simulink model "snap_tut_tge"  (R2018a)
settings: Solver=VariableStepDiscrete  StartTime=0.0  StopTime=50000  RelTol=1e-3
undefined symbols (not defined in the file): bad_frame, Bit, Both, bram, c, cnt_rst, core_rst, d, data, data_in, eof, eof_in, Falling, hex2dec, ip, ip_in, led, led_rx, led_tx, led_up, link_up, Location, Lower, Minimum_Area, notused, out, overrun, reg, Rising, ROACH2, sfp, SNAP, tx_full, tx_over, Unsigned, Upper, valid, valid_in, Width, xc7k160t
libraries: xbsIndex_r4 x1201, casper_library_misc x9, xps_library x5
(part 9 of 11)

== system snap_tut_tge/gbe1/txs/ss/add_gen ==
  note: Force MSbit of count to be '1' by negating busy as counter bit may be '0' or '1'
  note: A total count of bytes written to BRAM since trig
  note: Count of bytes in BRAM as well as done signal
  note: Do one capture by default
  note: prevent one extra write to address 0
  note: To storage
  vin : Inport
  din : Inport  Port=2
  we : Inport  Port=3
  go : Inport  Port=4
  cont : Inport  Port=5
  init : Inport  Port=6
  Concat : xbsIndex_r4/Concat  num_inputs=3  dbl_ovrd=off  block_type=concat
  Convert : xbsIndex_r4/Convert  gui_display_data_type=Fixed-point  arith_type=Unsigned  n_bits=32-nsamples-log2(increment)-1  bin_pt=0  float_type=Single  exp_bits=8  fraction_bits=24  quantization=Truncate  overflow=Wrap  en=off  latency=0  pipeline=off  dbl_ovrd=off  block_type=convert
  Delay{,3..6} (5 alike) : xbsIndex_r4/Delay  rst=off  infoeditControl=Selection of Reset will increase slice count due to use of real FFs and instead of SRLs  en=off  latency=1  reg_retiming=on  dbl_ovrd=off  block_type=delay
  Delay1 : xbsIndex_r4/Delay  rst=off  infoeditControl=Selection of Reset will increase slice count due to use of real FFs and instead of SRLs  en=off  latency=1  reg_retiming=off  dbl_ovrd=off  block_type=delay
  Delay2 : xbsIndex_r4/Delay  rst=off  infoeditControl=Selection of Reset will increase slice count due to use of real FFs and instead of SRLs  en=off  latency=1  reg_retiming=off  dbl_ovrd=off  block_type=delay
  Delay7 : xbsIndex_r4/Delay  rst=off  infoeditControl=Selection of Reset will increase slice count due to use of real FFs and instead of SRLs  en=off  latency=1  reg_retiming=off  dbl_ovrd=off  block_type=delay
  Inverter : xbsIndex_r4/Inverter  en=off  latency=1  dbl_ovrd=off  block_type=inv
  Inverter1 : xbsIndex_r4/Inverter  en=off  latency=0  dbl_ovrd=off  block_type=inv
  Logical1 : xbsIndex_r4/Logical  logical_function=AND  inputs=2  en=off  latency=1  precision=Full  arith_type=Unsigned  n_bits=8  bin_pt=2  align_bp=on  dbl_ovrd=off  block_type=logical
  Logical2 : xbsIndex_r4/Logical  logical_function=AND  inputs=2  en=off  latency=1  precision=Full  arith_type=Unsigned  n_bits=8  bin_pt=2  align_bp=on  dbl_ovrd=off  block_type=logical
  Logical4 : xbsIndex_r4/Logical  logical_function=OR  inputs=2  en=off  latency=0  precision=Full  arith_type=Unsigned  n_bits=8  bin_pt=2  align_bp=on  dbl_ovrd=off  block_type=logical
  Logical6 : xbsIndex_r4/Logical  logical_function=AND  inputs=3  en=off  latency=0  precision=Full  arith_type=Unsigned  n_bits=8  bin_pt=2  align_bp=on  dbl_ovrd=off  block_type=logical
  Register3 : xbsIndex_r4/Register  init=0  rst=on  en=on  dbl_ovrd=off  block_type=register
  Register4 : xbsIndex_r4/Register  init=0  rst=off  en=on  dbl_ovrd=off  block_type=register
  Register5 : xbsIndex_r4/Register  init=1  rst=on  en=on  dbl_ovrd=off  block_type=register
  Shift : xbsIndex_r4/Shift  shift_dir=Left  shift_bits=32-nsamples-log2(increment)-1-1  en=off  latency=1  precision=Full  arith_type="Signed  (2's comp)"  n_bits=16  bin_pt=14  quantization=Truncate  overflow=Wrap  dbl_ovrd=off  block_type=shift
  add_gen : xbsIndex_r4/Counter  cnt_type=Free Running  cnt_to=1  operation=Up  start_count=0  cnt_by_val=increment  arith_type=Unsigned  n_bits=counter_size  bin_pt=0  load_pin=off  rst=on  en=on  explicit_period=on  period=1  use_behavioral_HDL=off  implementation=DSP48  use_rpm=on  dbl_ovrd=off  block_type=counter
  edge_detect : Subsystem  AncestorBlock=casper_library_misc/edge_detect  mask(edge_detect){edge=Both, polarity=Active High, x_in=[0 0.08 0.08 0.16 0.16 0.24 0.24 0.32 0.32 0.4], y_in=[-1 -1  1  1  1  1 -1 -1 -1 -1], x_out=[0.6 0.68 0.68 0.76 0.76 0.84 0.84 0.92 0.92 1], y_out=[-1 -1  1  1 -1 -1  1  1 -1 -1]}
      mask prompts: edge "Edge Type"; polarity "Output Polarity"; x_in "Input X Positions"; y_in "Input Y Positions"; x_out "Output X Positions"; y_out "Output Y Positions"
      mask help: Output is active for one-cycle after each edge of the specified type (i.e. rising, falling or both).
      mask init:
      | edge_detect_init(gcb,...
      |     'edge',edge,...
      |     'polarity',polarity,...
      |     'x_in',x_in,...
      |     'x_out',x_out,...
      |     'y_in',y_in,...
      |     'y_out',y_out);
      | 
      | x_in_num=str2num(getfield(getfield(get_param(gcb,'UserData'),'parameters'),'x_in'));
      | x_out_num=str2num(getfield(getfield(get_param(gcb,'UserData'),'parameters'),'x_out'));
      | y_in_num=str2num(getfield(getfield(get_param(gcb,'UserData'),'parameters'),'y_in'));
      | y_out_num=str2num(getfield(getfield(get_param(gcb,'UserData'),'parameters'),'y_out'));
  edge_detect1 : Subsystem  AncestorBlock=casper_library_scopes/snapshot/add_gen/edge_detect  mask(edge_detect){edge=Both, polarity=Active High, x_in=[0 0.08 0.08 0.16 0.16 0.24 0.24 0.32 0.32 0.4], y_in=[-1 -1  1  1  1  1 -1 -1 -1 -1], x_out=[0.6 0.68 0.68 0.76 0.76 0.84 0.84 0.92 0.92 1], y_out=[-1 -1  1  1 -1 -1  1  1 -1 -1]}
      mask prompts: edge "Edge Type"; polarity "Output Polarity"; x_in "Input X Positions"; y_in "Input Y Positions"; x_out "Output X Positions"; y_out "Output Y Positions"
      mask help: Output is active for one-cycle after each edge of the specified type (i.e. rising, falling or both).
      mask init:
      | edge_detect_init(gcb,...
      |     'edge',edge,...
      |     'polarity',polarity,...
      |     'x_in',x_in,...
      |     'x_out',x_out,...
      |     'y_in',y_in,...
      |     'y_out',y_out);
      | 
      | x_in_num=str2num(getfield(getfield(get_param(gcb,'UserData'),'parameters'),'x_in'));
      | x_out_num=str2num(getfield(getfield(get_param(gcb,'UserData'),'parameters'),'x_out'));
      | y_in_num=str2num(getfield(getfield(get_param(gcb,'UserData'),'parameters'),'y_in'));
      | y_out_num=str2num(getfield(getfield(get_param(gcb,'UserData'),'parameters'),'y_out'));
  slice1 : xbsIndex_r4/Slice  nbits=nsamples+log2(increment)  boolean_output=off  mode=Lower Bit Location + Width  bit1=0  base1=LSB of Input  bit0=0  base0=LSB of Input  dbl_ovrd=off  block_type=slice
  slice2 : xbsIndex_r4/Slice  nbits=nsamples-burst_size  boolean_output=off  mode=Lower Bit Location + Width  bit1=0  base1=LSB of Input  bit0=log2(increment)+burst_size  base0=LSB of Input  dbl_ovrd=off  block_type=slice
  slice3 : xbsIndex_r4/Slice  nbits=1  boolean_output=on  mode=Lower Bit Location + Width  bit1=0  base1=MSB of Input  bit0=nsamples + log2(increment)  base0=LSB of Input  dbl_ovrd=off  block_type=slice
  vout : Outport
  add : Outport  Port=2
  dout : Outport  Port=3
  we_o : Outport  Port=4
  status : Outport  Port=5
  en_cnt : Outport  Port=6
  done : Outport  Port=7
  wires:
  Delay6/1 -> dout/1
  Delay5/1 -> Delay7/1
  Delay4/1 -> Delay/1, Register3/1, Register3/3, add_gen/1
  Delay3/1 -> Register5/1, Logical4/1
  Delay7/1 -> Register4/1
  Logical1/1 -> Logical6/3
  go/1 -> Logical1/2
  we/1 -> Logical1/1
  Logical4/1 -> Logical6/2
  Inverter/1 -> Concat/2
  slice1/1 -> Delay1/1
  Delay1/1 -> Concat/3
  din/1 -> Delay6/1
  Delay2/1 -> en_cnt/1
  slice2/1 -> add/1
  Convert/1 -> Shift/1
  Concat/1 -> status/1
  Logical6/1 -> add_gen/2, Register3/2, Logical2/1, we_o/1
  init/1 -> Delay4/1
  slice3/1 -> edge_detect/1(in)
  Register5/1 -> Logical6/1, edge_detect1/1(in), Inverter/1, Convert/1
  add_gen/1 -> slice3/1, Delay2/1, slice1/1, slice2/1
  vin/1 -> Delay5/1
  Register3/1 -> Logical2/2
  Logical2/1 -> Register4/2
  Register4/1 -> vout/1
  edge_detect/1(out) -> Register5/3, Inverter1/1
  cont/1 -> Delay3/1
  Inverter1/1 -> Logical4/2
  Delay/1 -> Register5/2
  Shift/1 -> Concat/1
  edge_detect1/1(out) -> done/1

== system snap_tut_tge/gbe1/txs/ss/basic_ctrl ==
  vin : Inport
  din : Inport  Port=2
  we : Inport  Port=3
  trig : Inport  Port=4
  ctrl : Inport  Port=5
  stopi : Inport  Port=6
  Constant : xbsIndex_r4/Constant  const=1  gui_display_data_type=Fixed-point  arith_type=Boolean  n_bits=16  bin_pt=14  preci_type=Single  exp_width=8  frac_width=24  explicit_period=on  period=1  equ=P=C  opselect=C  inp2=PCIN>>17  opr=+  inp1=P  carry=CIN  dbl_ovrd=off  block_type=constant
  Constant1 : xbsIndex_r4/Constant  const=1  gui_display_data_type=Fixed-point  arith_type=Boolean  n_bits=1  bin_pt=0  preci_type=Single  exp_width=8  frac_width=24  explicit_period=on  period=1  equ=P=C  opselect=C  inp2=PCIN>>17  opr=+  inp1=P  carry=CIN  dbl_ovrd=off  block_type=constant
  Constant2 : xbsIndex_r4/Constant  const=1  gui_display_data_type=Fixed-point  arith_type=Boolean  n_bits=1  bin_pt=0  preci_type=Single  exp_width=8  frac_width=24  explicit_period=on  period=1  equ=P=C  opselect=C  inp2=PCIN>>17  opr=+  inp1=P  carry=CIN  dbl_ovrd=off  block_type=constant
  Delay1 : xbsIndex_r4/Delay  rst=off  infoeditControl=Selection of Reset will increase slice count due to use of real FFs and instead of SRLs  en=off  latency=1  reg_retiming=off  dbl_ovrd=off  block_type=delay
  Delay2 : xbsIndex_r4/Delay  rst=off  infoeditControl=Selection of Reset will increase slice count due to use of real FFs and instead of SRLs  en=off  latency=1  reg_retiming=off  dbl_ovrd=off  block_type=delay
  Delay3 : xbsIndex_r4/Delay  rst=off  infoeditControl=Selection of Reset will increase slice count due to use of real FFs and instead of SRLs  en=off  latency=1  reg_retiming=off  dbl_ovrd=off  block_type=delay
  Inverter : xbsIndex_r4/Inverter  en=off  latency=0  dbl_ovrd=off  block_type=inv
  Logical : xbsIndex_r4/Logical  logical_function=AND  inputs=2  en=off  latency=0  precision=Full  arith_type=Unsigned  n_bits=16  bin_pt=0  align_bp=on  dbl_ovrd=off  block_type=logical
  Mux1 : xbsIndex_r4/Mux  inputs=2  en=off  latency=0  precision=Full  arith_type="Signed  (2's comp)"  n_bits=8  bin_pt=2  quantization=Truncate  overflow=Wrap  dbl_ovrd=off  block_type=mux
  Mux2 : xbsIndex_r4/Mux  inputs=2  en=off  latency=0  precision=Full  arith_type="Signed  (2's comp)"  n_bits=8  bin_pt=2  quantization=Truncate  overflow=Wrap  dbl_ovrd=off  block_type=mux
  Register1 : xbsIndex_r4/Register  init=0  rst=on  en=on  dbl_ovrd=off  block_type=register
  Register6 : xbsIndex_r4/Register  init=0  rst=on  en=on  dbl_ovrd=off  block_type=register
  dram_munge : Subsystem  mask{dram=off, data_width=data_width}
      mask prompts: data_width "data width"
      mask init:
      | set_param(gcb,'LinkStatus','inactive');
      | if strcmp(dram,'on'),
      |     set_param([gcb,'/dram'], 'const', '1');
      | else,
      |     set_param([gcb,'/dram'], 'const', '0');
      | end
      | set_param([gcb,'/data_choice'], ...
      |         'precision', 'User Defined', ...
      |         'arith_type', 'Unsigned', ...
      |         'n_bits', num2str(data_width), 'bin_pt', '0', ...
      |         'quantization', 'Truncate', ...
      |         'overflow', 'Wrap');
  edge_detect : casper_library_misc/edge_detect  edge=Rising  polarity=Active High  x_in=[0 0.08 0.08 0.16 0.16 0.24 0.24 0.32 0.32 0.4]  y_in="[-1 -1  1  1  1  1  1  1  1  1]"  x_out=[0.6 0.68 0.68 0.76 0.76 0.84 0.84 0.92 0.92 1]  y_out="[-1 -1  1  1 -1 -1 -1 -1 -1 -1]"
      link override Delay: sg_icon_stat=45,16,1,1,white,blue,0,07b98262,right,,[ ],[ ]  sg_mask_display=fprintf('','COMMENT: begin icon graphics'); patch([0 45 45 0 0 ],[0 0 16 16 0 ],[0.77 0.82 0.91 ]); plot([0 45 45 0 0 ],[0 0 16 16 0 ]); patch([17.55 20.44 22.44 24.44 26.44 22.44 19.55 17.55 ],[10.22 10.22 12.22 10.22 12.22 12.22 12.22 10.22 ],[1 1 1 ]); patch([19.55 22.44 20.44 17.55 19.55 ],[8.22 8.22 10.22 10.22 8.22 ],[0.931 0.946 0.973 ]); patch([17.55 20.44 22.44 19.55 17.55 ],[6.22 6.22 8.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
      link override Inverter: sg_icon_stat=45,16,1,1,white,blue,0,267846e5,right,,[ ],[ ]  sg_mask_display=fprintf('','COMMENT: begin icon graphics'); patch([0 45 45 0 0 ],[0 0 16 16 0 ],[0.77 0.82 0.91 ]); plot([0 45 45 0 0 ],[0 0 16 16 0 ]); patch([17.55 20.44 22.44 24.44 26.44 22.44 19.55 17.55 ],[10.22 10.22 12.22 10.22 12.22 12.22 12.22 10.22 ],[1 1 1 ]); patch([19.55 22.44 20.44 17.55 19.55 ],[8.22 8.22 10.22 10.22 8.22 ],[0.931 0.946 0.973 ]); patch([17.55 20.44 22.44 19.55 17.55 ],[6.22 6.22 8.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
      link override edge_op: sg_icon_stat=45,44,2,1,white,blue,0,affe8783,right,,[ ],[ ]  sg_mask_display=fprintf('','COMMENT: begin icon graphics'); patch([0 45 45 0 0 ],[0 0 44 44 0 ],[0.77 0.82 0.91 ]); plot([0 45 45 0 0 ],[0 0 44 44 0 ]); patch([8.65 17.32 23.32 29.32 35.32 23.32 14.65 8.65 ],[28.66 28.66 34.66 28.66 34.66 34.66 34.66 28.66 ],[1 1 1 ]); patch([14.65 23.32 17.32 8.65 14.65 ],[22.66 22.66 28.66 28.66 22.66 ],[0.931 0.946 0.973 ]); patch([8.65 17.32 23.32 14.65 8.65 ],[16.66 16.66 22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
  enable : xbsIndex_r4/Slice  nbits=1  boolean_output=on  mode=Lower Bit Location + Width  bit1=0  base1=LSB of Input  bit0=0  base0=LSB of Input  dbl_ovrd=off  block_type=slice
  trig_src : xbsIndex_r4/Slice  nbits=1  boolean_output=on  mode=Lower Bit Location + Width  bit1=0  base1=LSB of Input  bit0=1  base0=LSB of Input  dbl_ovrd=off  block_type=slice
  valid_src : xbsIndex_r4/Slice  nbits=1  boolean_output=on  mode=Lower Bit Location + Width  bit1=0  base1=LSB of Input  bit0=2  base0=LSB of Input  dbl_ovrd=off  block_type=slice
  vout : Outport
  dout : Outport  Port=2
  we_o : Outport  Port=3
  go : Outport  Port=4
  stop : Outport  Port=5
  init : Outport  Port=6
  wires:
  Delay1/1 -> edge_detect/1
  Delay3/1 -> Mux1/1
  Delay2/1 -> Mux2/1
  dram_munge/1(vout) -> vout/1
  vin/1 -> dram_munge/1(vin)
  dram_munge/3(we_o) -> we_o/1
  dram_munge/2(dout) -> dout/1
  din/1 -> dram_munge/2(din)
  Inverter/1 -> Logical/2
  Mux2/1 -> Logical/1, Register6/1
  Register6/1 -> go/1
  trig/1 -> Mux2/2
  Mux1/1 -> dram_munge/3(we)
  we/1 -> Mux1/2
  ctrl/1 -> enable/1, valid_src/1, trig_src/1
  edge_detect/1 -> Inverter/1, Register1/3, dram_munge/4(init), Register6/2, init/1
  enable/1 -> Delay1/1
  Constant1/1 -> Mux2/3
  Constant2/1 -> Mux1/3
  trig_src/1 -> Delay2/1
  valid_src/1 -> Delay3/1
  Constant/1 -> Register1/1
  Register1/1 -> Register6/3
  Logical/1 -> Register1/2
  stopi/1 -> stop/1

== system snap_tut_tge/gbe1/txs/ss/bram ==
  addr : Inport
  data_in : Inport  Port=2
  we : Inport  Port=3
  Terminator : Terminator
  Terminator1 : Terminator
  Terminator2 : Terminator
  calc_add : Subsystem  mask{data_width=128, addr_width=13, sample_rate=sample_rate}
      mask prompts: data_width "data width"; addr_width "address width"; sample_rate "sample rate"
  convert_addr : xbsIndex_r4/Convert  gui_display_data_type=Fixed-point  arith_type=Unsigned  n_bits=addr_width  bin_pt=0  float_type=Single  exp_bits=8  fraction_bits=24  quantization=Truncate  overflow=Wrap  en=off  latency=0  pipeline=off  dbl_ovrd=off  block_type=convert
  convert_din1 : xbsIndex_r4/Convert  gui_display_data_type=Fixed-point  arith_type=Unsigned  n_bits=128  bin_pt=0  float_type=Single  exp_bits=8  fraction_bits=24  quantization=Truncate  overflow=Wrap  en=off  latency=0  pipeline=off  dbl_ovrd=off  block_type=convert
  convert_we : xbsIndex_r4/Convert  gui_display_data_type=Fixed-point  arith_type=Unsigned  n_bits=1  bin_pt=0  float_type=Single  exp_bits=8  fraction_bits=24  quantization=Truncate  overflow=Wrap  en=off  latency=0  pipeline=off  dbl_ovrd=off  block_type=convert
  munge_in : Subsystem  AncestorBlock=casper_library_flow_control/munge  mask(munge){divisions=4, div_size=[32 32 32 32], order=[3  2  1  0], arith_type_out=Unsigned, bin_pt_out=0}
      mask prompts: divisions "Number of divisions"; div_size "Division size (bits)"; order "Division packing order"; arith_type_out "Output arithmetic type"; bin_pt_out "Output binary point"
      mask help: Splits an input bus into the specified number of divisions and then recombines them in the order specified (most significant division = 0,least = number divisions-1)
      mask init:
      | munge_init(gcb, ...
      |     'divisions', divisions, ...
      |     'div_size', div_size, ...
      |     'order', order, ...
      |     'arith_type_out', arith_type_out, ...
      |     'bin_pt_out', bin_pt_out);
  munge_out : Subsystem  AncestorBlock=casper_library_flow_control/munge  mask(munge){divisions=4, div_size=[32 32 32 32], order=[3  2  1  0], arith_type_out=Unsigned, bin_pt_out=0}
      mask prompts: divisions "Number of divisions"; div_size "Division size (bits)"; order "Division packing order"; arith_type_out "Output arithmetic type"; bin_pt_out "Output binary point"
      mask help: Splits an input bus into the specified number of divisions and then recombines them in the order specified (most significant division = 0,least = number divisions-1)
      mask init:
      | munge_init(gcb, ...
      |     'divisions', divisions, ...
      |     'div_size', div_size, ...
      |     'order', order, ...
      |     'arith_type_out', arith_type_out, ...
      |     'bin_pt_out', bin_pt_out);
  sim_mem : Subsystem  mask{arith_type=Unsigned, addr_width=13, data_width=128, data_bin_pt=0, init_vals=[0     1     2     3     4     5     6     7     8     9    10    11    12    13    14    15    16    17    18    19    20    21    22    23    24    25    26    27    28    29    30    31    32    33    34    35    36    37    38    39    40    41    42    43    44    45    46    47    48    49    50    51    52    53    54    55    56    57    58    59    60    61    62    63    64    65    66  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, sample_rate=1, csp_latency=1}
      mask prompts: arith_type "Output Data Type"; addr_width "Address width"; data_width "Data width"; data_bin_pt "Data Binary Point"; init_vals "Initial values"; sample_rate "Sample rate"; csp_latency "Latency"
      mask init:
      | % set_param([gcb, '/data_to_xilinx'], 'arith_type', arith_type)
      | % set_param([gcb, '/data_to_xilinx'], 'n_bits', get_param(gcb, 'data_width'))
  snap_tut_tge_gbe1_txs_ss_bram_addr : xbsIndex_r4/Gateway Out  inherit_from_input=off  hdl_port=on  rows=1  columns=1  UseAsDAC=off  DACChannel='1'  interface=None  automatic_assignment=on  address_offset=hex2dec('00')  intf_name=''  intf_description=''  timing_constraint=None  locs_specified=off  LOCs={'A5','B9','A9','C1','A3','G6','E9','A6','A7','A8','B8','B1','B3','D9','B5','B4','B6','C2'}  io_standard={}  block_type=gatewayout
  snap_tut_tge_gbe1_txs_ss_bram_data_in : xbsIndex_r4/Gateway Out  inherit_from_input=off  hdl_port=on  rows=1  columns=1  UseAsDAC=off  DACChannel='1'  interface=None  automatic_assignment=on  address_offset=hex2dec('00')  intf_name=''  intf_description=''  timing_constraint=None  locs_specified=off  LOCs={'B21','B22','A22','B23','B19','C19','A20','A21','A23','B24','A24','A25','E18','D18','C18','B18'}  io_standard={}  block_type=gatewayout
  snap_tut_tge_gbe1_txs_ss_bram_data_out : xbsIndex_r4/Gateway In  gui_display_data_type=Fixed-point  arith_type=Unsigned  n_bits=128  bin_pt=0  preci_type=Single  exp_width=8  frac_width=24  rows=1  columns=1  quantization=Truncate  overflow=Wrap  period=sample_rate  UseAsADC=off  ADCChannel='1'  interface=None  automatic_assignment=on  address_offset=hex2dec('00')  intf_name=''  intf_description=''  default_value=0  timing_constraint=None  locs_specified=off  LOCs={}  io_standard={}  inherit_from_input=off  hdl_port=on  dbl_ovrd=off  block_type=gatewayin
  snap_tut_tge_gbe1_txs_ss_bram_we : xbsIndex_r4/Gateway Out  inherit_from_input=off  hdl_port=on  rows=1  columns=1  UseAsDAC=off  DACChannel='1'  interface=None  automatic_assignment=on  address_offset=hex2dec('00')  intf_name=''  intf_description=''  timing_constraint=None  locs_specified=off  LOCs={'A14'}  io_standard={}  block_type=gatewayout
  data_out : Outport
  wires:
  munge_in/1(dout) -> convert_din1/1, sim_mem/2(data)
  we/1 -> convert_we/1, sim_mem/3(we)
  addr/1 -> calc_add/1(in)
  convert_we/1 -> snap_tut_tge_gbe1_txs_ss_bram_we/1
  snap_tut_tge_gbe1_txs_ss_bram_addr/1 -> Terminator/1
  snap_tut_tge_gbe1_txs_ss_bram_data_in/1 -> Terminator1/1
  snap_tut_tge_gbe1_txs_ss_bram_we/1 -> Terminator2/1
  calc_add/1(out) -> convert_addr/1, sim_mem/1(addr)
  data_in/1 -> munge_in/1(din)
  convert_din1/1 -> snap_tut_tge_gbe1_txs_ss_bram_data_in/1
  convert_addr/1 -> snap_tut_tge_gbe1_txs_ss_bram_addr/1
  snap_tut_tge_gbe1_txs_ss_bram_data_out/1 -> munge_out/1(din)
  sim_mem/1(data_out) -> snap_tut_tge_gbe1_txs_ss_bram_data_out/1
  munge_out/1(dout) -> data_out/1

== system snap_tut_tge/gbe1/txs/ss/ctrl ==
  convert1_1 : DataTypeConversion  OutDataTypeStr=fixdt('ufix32_En0')
  convert2_1 : DataTypeConversion  OutDataTypeStr=fixdt('ufix32_En0')  ConvertRealWorld=Stored Integer (SI)
  gain_1 : Gain
  io_delay : xbsIndex_r4/Delay  rst=off  infoeditControl=Selection of Reset will increase slice count due to use of real FFs and instead of SRLs  en=off  latency=0  reg_retiming=on  dbl_ovrd=off  block_type=delay
  reint1 : xbsIndex_r4/Reinterpret  force_arith_type=on  arith_type=Unsigned  force_bin_pt=on  bin_pt=0  block_type=reinterpret
  sim_1 : Constant  Value=0
  slice_reg : xbsIndex_r4/Slice  nbits=32  boolean_output=off  mode=Lower Bit Location + Width  bit1=0  base1=MSB of Input  bit0=0  base0=LSB of Input  dbl_ovrd=off  block_type=slice
  snap_tut_tge_gbe1_txs_ss_ctrl_user_data_out : xbsIndex_r4/Gateway In  gui_display_data_type=Fixed-point  arith_type=Unsigned  n_bits=32  bin_pt=0  preci_type=Single  exp_width=8  frac_width=24  rows=1  columns=1  quantization="Round  (unbiased: +/- Inf)"  overflow=Saturate  period=1  UseAsADC=off  ADCChannel='1'  interface=None  automatic_assignment=on  address_offset=hex2dec('00')  intf_name=''  intf_description=''  default_value=0  timing_constraint=None  locs_specified=off  LOCs={}  io_standard={}  inherit_from_input=off  hdl_port=on  dbl_ovrd=off  block_type=gatewayin
  in_reg : Outport
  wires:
  snap_tut_tge_gbe1_txs_ss_ctrl_user_data_out/1 -> io_delay/1
  sim_1/1 -> convert1_1/1
  convert1_1/1 -> convert2_1/1
  convert2_1/1 -> gain_1/1
  gain_1/1 -> snap_tut_tge_gbe1_txs_ss_ctrl_user_data_out/1
  io_delay/1 -> slice_reg/1
  slice_reg/1 -> reint1/1
  reint1/1 -> in_reg/1

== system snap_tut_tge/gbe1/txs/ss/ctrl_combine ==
  in1 : Inport
  in2 : Inport  Port=2
  in3 : Inport  Port=3
  in4 : Inport  Port=4
  concatenate : xbsIndex_r4/Concat  num_inputs=4  dbl_ovrd=off  block_type=concat
  reinterpret{1..4} (4 alike) : xbsIndex_r4/Reinterpret  force_arith_type=on  arith_type=Unsigned  force_bin_pt=on  bin_pt=0  block_type=reinterpret
  bus_out : Outport
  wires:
  concatenate/1 -> bus_out/1
  in1/1 -> reinterpret1/1
  reinterpret1/1 -> concatenate/1
  in2/1 -> reinterpret2/1
  reinterpret2/1 -> concatenate/2
  in3/1 -> reinterpret3/1
  reinterpret3/1 -> concatenate/3
  in4/1 -> reinterpret4/1
  reinterpret4/1 -> concatenate/4

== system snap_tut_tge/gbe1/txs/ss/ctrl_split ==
  bus_in : Inport
  reinterpret2 : xbsIndex_r4/Reinterpret  force_arith_type=on  arith_type=Unsigned  force_bin_pt=on  bin_pt=0  block_type=reinterpret
  reinterpret4 : xbsIndex_r4/Reinterpret  force_arith_type=on  arith_type=Unsigned  force_bin_pt=on  bin_pt=0  block_type=reinterpret
  slice1 : xbsIndex_r4/Slice  nbits=1  boolean_output=on  mode=Upper Bit Location + Width  bit1=-31  base1=MSB of Input  bit0=0  base0=LSB of Input  dbl_ovrd=off  block_type=slice
  slice2 : xbsIndex_r4/Slice  nbits=2  boolean_output=off  mode=Upper Bit Location + Width  bit1=-29  base1=MSB of Input  bit0=0  base0=LSB of Input  dbl_ovrd=off  block_type=slice
  slice3 : xbsIndex_r4/Slice  nbits=1  boolean_output=on  mode=Upper Bit Location + Width  bit1=-28  base1=MSB of Input  bit0=0  base0=LSB of Input  dbl_ovrd=off  block_type=slice
  slice4 : xbsIndex_r4/Slice  nbits=28  boolean_output=off  mode=Upper Bit Location + Width  bit1=0  base1=MSB of Input  bit0=0  base0=LSB of Input  dbl_ovrd=off  block_type=slice
  msb_out4 : Outport
  out3 : Outport  Port=2
  out2 : Outport  Port=3
  lsb_out1 : Outport  Port=4
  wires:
  bus_in/1 -> slice4/1, slice3/1, slice2/1, slice1/1
  slice4/1 -> reinterpret4/1
  reinterpret4/1 -> msb_out4/1
  slice3/1 -> out3/1
  slice2/1 -> reinterpret2/1
  reinterpret2/1 -> out2/1
  slice1/1 -> lsb_out1/1

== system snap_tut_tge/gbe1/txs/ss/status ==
  out_reg : Inport
  assert_reg : xbsIndex_r4/Assert  assert_type=on  type_source=Explicitly  gui_display_data_type=Fixed-point  arith_type=Unsigned  n_bits=32  bin_pt=0  preci_type=Single  exp_width=8  frac_width=24  assert_rate=off  rate_source=Explicitly  period=1  output_port=on  block_type=assert
  cast_gw : xbsIndex_r4/Convert  gui_display_data_type=Fixed-point  arith_type=Unsigned  n_bits=32  bin_pt=0  float_type=Single  exp_bits=8  fraction_bits=24  quantization=Truncate  overflow=Wrap  en=off  latency=1  pipeline=off  dbl_ovrd=off  block_type=convert
  io_delay : xbsIndex_r4/Delay  rst=off  infoeditControl=Selection of Reset will increase slice count due to use of real FFs and instead of SRLs  en=off  latency=0  reg_retiming=on  dbl_ovrd=off  block_type=delay
  reint1 : xbsIndex_r4/Reinterpret  force_arith_type=on  arith_type=Unsigned  force_bin_pt=on  bin_pt=0  block_type=reinterpret
  sim_out : Terminator
  snap_tut_tge_gbe1_txs_ss_status_user_data_in : xbsIndex_r4/Gateway Out  inherit_from_input=off  hdl_port=on  rows=1  columns=1  UseAsDAC=off  DACChannel='1'  interface=None  automatic_assignment=on  address_offset=hex2dec('00')  intf_name=''  intf_description=''  timing_constraint=None  locs_specified=off  LOCs={}  io_standard={}  block_type=gatewayout
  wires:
  io_delay/1 -> cast_gw/1
  cast_gw/1 -> snap_tut_tge_gbe1_txs_ss_status_user_data_in/1
  snap_tut_tge_gbe1_txs_ss_status_user_data_in/1 -> sim_out/1
  out_reg/1 -> assert_reg/1
  assert_reg/1 -> reint1/1
  reint1/1 -> io_delay/1

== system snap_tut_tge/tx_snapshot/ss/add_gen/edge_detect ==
  in : Inport
  Delay : xbsIndex_r4/Delay  rst=off  infoeditControl=Selection of Reset will increase slice count due to use of real FFs and instead of SRLs  en=off  latency=1  reg_retiming=off  dbl_ovrd=off  block_type=delay
  Inverter : xbsIndex_r4/Inverter  en=off  latency=0  dbl_ovrd=off  block_type=inv
  edge_op : xbsIndex_r4/Logical  logical_function=XNOR  inputs=2  en=off  latency=0  precision=Full  arith_type=Unsigned  n_bits=8  bin_pt=2  align_bp=on  dbl_ovrd=off  block_type=logical
  out : Outport
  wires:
  Delay/1 -> edge_op/2
  in/1 -> Delay/1, Inverter/1
  edge_op/1 -> out/1
  Inverter/1 -> edge_op/1

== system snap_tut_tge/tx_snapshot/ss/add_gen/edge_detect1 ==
  in : Inport
  Delay : xbsIndex_r4/Delay  rst=off  infoeditControl=Selection of Reset will increase slice count due to use of real FFs and instead of SRLs  en=off  latency=1  reg_retiming=off  dbl_ovrd=off  block_type=delay
  Inverter : xbsIndex_r4/Inverter  en=off  latency=0  dbl_ovrd=off  block_type=inv
  edge_op : xbsIndex_r4/Logical  logical_function=XNOR  inputs=2  en=off  latency=0  precision=Full  arith_type=Unsigned  n_bits=8  bin_pt=2  align_bp=on  dbl_ovrd=off  block_type=logical
  out : Outport
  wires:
  Inverter/1 -> edge_op/1
  edge_op/1 -> out/1
  in/1 -> Inverter/1, Delay/1
  Delay/1 -> edge_op/2

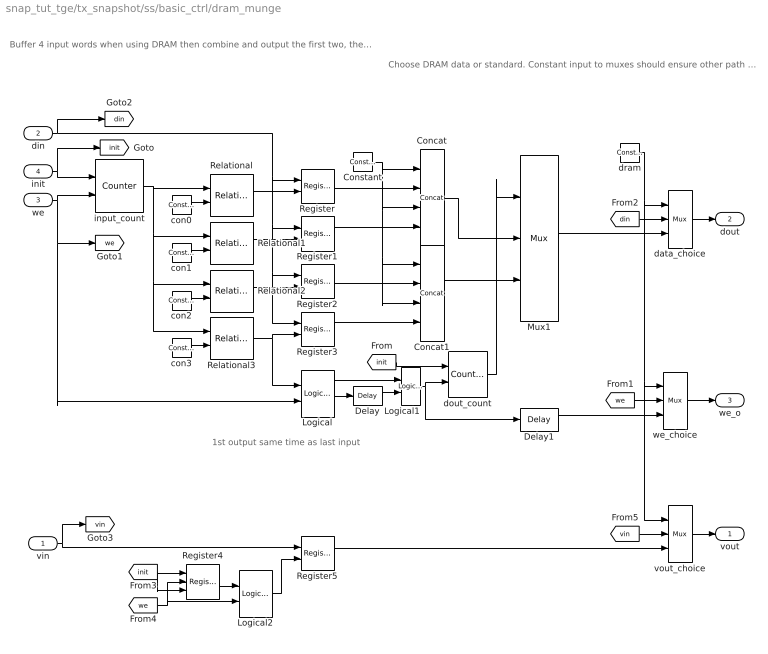
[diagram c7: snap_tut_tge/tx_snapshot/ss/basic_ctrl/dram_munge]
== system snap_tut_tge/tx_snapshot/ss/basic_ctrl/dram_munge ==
  note: 1st output same time as last input
  note: Choose DRAM data or standard. Constant input to muxes should ensure other path optimised away
  note: Buffer 4 input words when using DRAM then combine and output the first two, then second. Ensures that a full burst goes through every time so that status register records number of bytes fully in DRAM
  vin : Inport
  din : Inport  Port=2
  we : Inport  Port=3
  init : Inport  Port=4
  Concat : xbsIndex_r4/Concat  num_inputs=4  dbl_ovrd=off  block_type=concat
  Concat1 : xbsIndex_r4/Concat  num_inputs=4  dbl_ovrd=off  block_type=concat
  Constant : xbsIndex_r4/Constant  const=0  gui_display_data_type=Fixed-point  arith_type=Unsigned  n_bits=8  bin_pt=0  preci_type=Single  exp_width=8  frac_width=24  explicit_period=on  period=1  equ=P=C  opselect=C  inp2=PCIN>>17  opr=+  inp1=P  carry=CIN  dbl_ovrd=off  block_type=constant
  Delay : xbsIndex_r4/Delay  rst=off  infoeditControl=Selection of Reset will increase slice count due to use of real FFs and instead of SRLs  en=off  latency=1  reg_retiming=off  dbl_ovrd=off  block_type=delay
  Delay1 : xbsIndex_r4/Delay  rst=off  infoeditControl=Selection of Reset will increase slice count due to use of real FFs and instead of SRLs  en=off  latency=1  reg_retiming=off  dbl_ovrd=off  block_type=delay
  Logical : xbsIndex_r4/Logical  logical_function=AND  inputs=2  en=off  latency=1  precision=Full  arith_type=Unsigned  n_bits=16  bin_pt=0  align_bp=on  dbl_ovrd=off  block_type=logical
  Logical1 : xbsIndex_r4/Logical  logical_function=OR  inputs=2  en=off  latency=0  precision=Full  arith_type=Unsigned  n_bits=16  bin_pt=0  align_bp=on  dbl_ovrd=off  block_type=logical
  Logical2 : xbsIndex_r4/Logical  logical_function=AND  inputs=2  en=off  latency=0  precision=Full  arith_type=Unsigned  n_bits=16  bin_pt=0  align_bp=on  dbl_ovrd=off  block_type=logical
  Mux1 : xbsIndex_r4/Mux  inputs=2  en=off  latency=1  precision=Full  arith_type=Unsigned  n_bits=16  bin_pt=14  quantization=Truncate  overflow=Wrap  dbl_ovrd=off  block_type=mux
  Register{,1..3,5} (5 alike) : xbsIndex_r4/Register  init=0  rst=off  en=on  dbl_ovrd=off  block_type=register
  Register4 : xbsIndex_r4/Register  init=0  rst=on  en=on  dbl_ovrd=off  block_type=register
  Relational{,1..3} (4 alike) : xbsIndex_r4/Relational  mode=a=b  op_type=Bool  en=off  latency=0  dbl_ovrd=off  block_type=relational
  con0 : xbsIndex_r4/Constant  const=0  gui_display_data_type=Fixed-point  arith_type=Unsigned  n_bits=2  bin_pt=0  preci_type=Single  exp_width=8  frac_width=24  explicit_period=on  period=1  equ=P=C  opselect=C  inp2=PCIN>>17  opr=+  inp1=P  carry=CIN  dbl_ovrd=off  block_type=constant
  con1 : xbsIndex_r4/Constant  const=1  gui_display_data_type=Fixed-point  arith_type=Unsigned  n_bits=2  bin_pt=0  preci_type=Single  exp_width=8  frac_width=24  explicit_period=on  period=1  equ=P=C  opselect=C  inp2=PCIN>>17  opr=+  inp1=P  carry=CIN  dbl_ovrd=off  block_type=constant
  con2 : xbsIndex_r4/Constant  const=2  gui_display_data_type=Fixed-point  arith_type=Unsigned  n_bits=2  bin_pt=0  preci_type=Single  exp_width=8  frac_width=24  explicit_period=on  period=1  equ=P=C  opselect=C  inp2=PCIN>>17  opr=+  inp1=P  carry=CIN  dbl_ovrd=off  block_type=constant
  con3 : xbsIndex_r4/Constant  const=3  gui_display_data_type=Fixed-point  arith_type=Unsigned  n_bits=2  bin_pt=0  preci_type=Single  exp_width=8  frac_width=24  explicit_period=on  period=1  equ=P=C  opselect=C  inp2=PCIN>>17  opr=+  inp1=P  carry=CIN  dbl_ovrd=off  block_type=constant
  data_choice : xbsIndex_r4/Mux  inputs=2  en=off  latency=0  precision=User Defined  arith_type=Unsigned  n_bits=128  bin_pt=0  quantization=Truncate  overflow=Wrap  dbl_ovrd=off  block_type=mux
  dout_count : xbsIndex_r4/Counter  cnt_type=Free Running  cnt_to=Inf  operation=Up  start_count=0  cnt_by_val=1  arith_type=Unsigned  n_bits=1  bin_pt=0  load_pin=off  rst=on  en=on  explicit_period=on  period=1  use_behavioral_HDL=off  implementation=Fabric  dbl_ovrd=off  block_type=counter
  dram : xbsIndex_r4/Constant  const=0  gui_display_data_type=Fixed-point  arith_type=Boolean  n_bits=16  bin_pt=14  preci_type=Single  exp_width=8  frac_width=24  explicit_period=on  period=1  equ=P=C  opselect=C  inp2=PCIN>>17  opr=+  inp1=P  carry=CIN  dbl_ovrd=off  block_type=constant
  input_count : xbsIndex_r4/Counter  cnt_type=Free Running  cnt_to=Inf  operation=Up  start_count=0  cnt_by_val=1  arith_type=Unsigned  n_bits=2  bin_pt=0  load_pin=off  rst=on  en=on  explicit_period=on  period=1  use_behavioral_HDL=off  implementation=Fabric  dbl_ovrd=off  block_type=counter
  vout_choice : xbsIndex_r4/Mux  inputs=2  en=off  latency=0  precision=Full  arith_type=Unsigned  n_bits=16  bin_pt=14  quantization=Truncate  overflow=Wrap  dbl_ovrd=off  block_type=mux
  we_choice : xbsIndex_r4/Mux  inputs=2  en=off  latency=0  precision=Full  arith_type=Unsigned  n_bits=16  bin_pt=14  quantization=Truncate  overflow=Wrap  dbl_ovrd=off  block_type=mux
  vout : Outport
  dout : Outport  Port=2
  we_o : Outport  Port=3
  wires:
  Register3/1 -> Concat1/4
  Register2/1 -> Concat1/2
  Constant/1 -> Concat1/3, Concat1/1, Concat/3, Concat/1
  Register1/1 -> Concat/4
  Register/1 -> Concat/2
  [vin] -> vout_choice/2
  Register5/1 -> vout_choice/3
  vout_choice/1 -> vout/1
  Logical2/1 -> Register5/2
  [we] -> Logical2/2, Register4/2
  vin/1 -> [vin], Register5/1
  Register4/1 -> Logical2/1
  [init] -> Register4/3, Register4/1
  dram/1 -> vout_choice/1, we_choice/1, data_choice/1
  [din] -> data_choice/2
  Mux1/1 -> data_choice/3
  [we] -> we_choice/2
  Delay1/1 -> we_choice/3
  we_choice/1 -> we_o/1
  dout_count/1 -> Mux1/1
  [init] -> dout_count/1
  Logical1/1 -> Delay1/1, dout_count/2
  Concat1/1 -> Mux1/3
  Concat/1 -> Mux1/2
  Delay/1 -> Logical1/2
  Logical/1 -> Logical1/1, Delay/1
  Relational3/1 -> Logical/1, Register3/2
  Relational2/1 -> Register2/2
  Relational1/1 -> Register1/2
  Relational/1 -> Register/2
  con3/1 -> Relational3/2
  con2/1 -> Relational2/2
  con1/1 -> Relational1/2
  con0/1 -> Relational/2
  input_count/1 -> Relational3/1, Relational2/1, Relational1/1, Relational/1
  din/1 -> [din], Register3/1, Register2/1, Register1/1, Register/1
  we/1 -> [we], Logical/2, input_count/2
  init/1 -> [init], input_count/1
  data_choice/1 -> dout/1

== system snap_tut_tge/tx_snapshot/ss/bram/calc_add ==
  note: If reading/writing words smaller than 32 bits, change address so that addressing is big endian instead of little, otherwise pass through
  note: Use behavioural HDL so that gets optimised to minimum logic
  in : Inport
  add_sub : xbsIndex_r4/AddSub  mode=Subtraction  use_carryin=off  use_carryout=off  en=off  latency=0  precision=User Defined  arith_type=Unsigned  n_bits=max(1, log2(32/data_width))  bin_pt=0  quantization=Truncate  overflow=Wrap  use_behavioral_HDL=on  hw_selection=Fabric  pipelined=off  dbl_ovrd=off  block_type=addsub
  concat : xbsIndex_r4/Concat  num_inputs=2  dbl_ovrd=off  block_type=concat
  const : xbsIndex_r4/Constant  const=max(0, 32/data_width-1)  gui_display_data_type=Fixed-point  arith_type=Unsigned  n_bits=max(1, log2(32/data_width))  bin_pt=0  preci_type=Single  exp_width=8  frac_width=24  explicit_period=on  period=sample_rate  equ=P=C  opselect=C  inp2=PCIN>>17  opr=+  inp1=P  carry=CIN  dbl_ovrd=off  block_type=constant
  convert_addr : xbsIndex_r4/Convert  gui_display_data_type=Fixed-point  arith_type=Unsigned  n_bits=addr_width  bin_pt=0  float_type=Single  exp_bits=8  fraction_bits=24  quantization=Truncate  overflow=Wrap  en=off  latency=0  pipeline=off  dbl_ovrd=off  block_type=convert
  lsw : xbsIndex_r4/Slice  nbits=max(1, log2(32/data_width))  boolean_output=off  mode=Lower Bit Location + Width  bit1=0  base1=MSB of Input  bit0=0  base0=LSB of Input  dbl_ovrd=off  block_type=slice
  manipulate : xbsIndex_r4/Constant  const=min(1, floor(32/data_width) - 1)  gui_display_data_type=Fixed-point  arith_type=Unsigned  n_bits=1  bin_pt=0  preci_type=Single  exp_width=8  frac_width=24  explicit_period=on  period=sample_rate  equ=P=C  opselect=C  inp2=PCIN>>17  opr=+  inp1=P  carry=CIN  dbl_ovrd=off  block_type=constant
  msw : xbsIndex_r4/Slice  nbits=addr_width - max(1, log2(32/data_width))  boolean_output=off  mode=Upper Bit Location + Width  bit1=0  base1=MSB of Input  bit0=0  base0=LSB of Input  dbl_ovrd=off  block_type=slice
  mux : xbsIndex_r4/Mux  inputs=2  en=off  latency=0  precision=Full  arith_type=Unsigned  n_bits=16  bin_pt=14  quantization=Truncate  overflow=Wrap  dbl_ovrd=off  block_type=mux
  out : Outport
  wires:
  in/1 -> convert_addr/1
  add_sub/1 -> concat/2
  msw/1 -> concat/1
  concat/1 -> mux/3
  manipulate/1 -> mux/1
  mux/1 -> out/1
  lsw/1 -> add_sub/2
  const/1 -> add_sub/1
  convert_addr/1 -> lsw/1, msw/1, mux/2

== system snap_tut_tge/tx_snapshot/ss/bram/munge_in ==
  din : Inport
  join : Subsystem  AncestorBlock=casper_library_flow_control/bus_create  mask(bus_create){inputNum=4}
      mask prompts: inputNum "Number of inputs:"
      mask init:
      | bus_create_init(gcb,...
      |     'inputNum', inputNum);
  reinterpret : xbsIndex_r4/Reinterpret  force_arith_type=on  arith_type=Unsigned  force_bin_pt=on  bin_pt=0  block_type=reinterpret
  reinterpret_out : xbsIndex_r4/Reinterpret  force_arith_type=on  arith_type=Unsigned  force_bin_pt=on  bin_pt=0  block_type=reinterpret
  split : Subsystem  AncestorBlock=casper_library_flow_control/bus_expand  mask(bus_expand){mode=divisions of arbitrary size, outputNum=1, outputWidth=[32 32 32 32], outputBinaryPt=[0 0 0 0], outputArithmeticType=[0 0 0 0], show_format=off, outputToWorkspace=off, variablePrefix=out, outputToModelAsWell=on}
      mask prompts: outputNum "Number of outputs:"; outputWidth "Output width [msb ... lsb]:"; outputBinaryPt "Output binary point position [msb ... lsb]:"; outputArithmeticType "Output arithmetic type (ufix=0, fix=1, bool=2) [msb ... lsb]:"; show_format "Print format string?"; outputToWorkspace "Output to workspace?"; variablePrefix "Variable name prefix:"; outputToModelAsWell "Output to model as well?"
      mask help: Expands a 'bus' made using a bus_create or Xilinx concat block. The input will be divided into the specified number of outputs with the specified arithmetic types. Divisions are made from most significant bit.
      mask init:
      | bus_expand_init(gcb,...
      |     'mode', mode, ...
      |     'outputNum', outputNum, ...
      |     'outputWidth', outputWidth, ...
      |     'outputBinaryPt', outputBinaryPt, ...
      |     'outputArithmeticType', outputArithmeticType, ...
      |     'show_format', show_format, ...
      |     'outputToWorkspace', outputToWorkspace, ...
      |     'variablePrefix', variablePrefix, ...
      |     'outputToModelAsWell', outputToModelAsWell);
  dout : Outport
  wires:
  reinterpret_out/1 -> dout/1
  din/1 -> reinterpret/1
  reinterpret/1 -> split/1(bus_in)
  join/1(bus_out) -> reinterpret_out/1
  split/4(lsb_out1) -> join/1(in1)
  split/3(out2) -> join/2(in2)
  split/2(out3) -> join/3(in3)
  split/1(msb_out4) -> join/4(in4)

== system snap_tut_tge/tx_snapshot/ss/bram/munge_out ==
  din : Inport
  join : Subsystem  AncestorBlock=casper_library_flow_control/bus_create  mask(bus_create){inputNum=4}
      mask prompts: inputNum "Number of inputs:"
      mask init:
      | bus_create_init(gcb,...
      |     'inputNum', inputNum);
  reinterpret : xbsIndex_r4/Reinterpret  force_arith_type=on  arith_type=Unsigned  force_bin_pt=on  bin_pt=0  block_type=reinterpret
  reinterpret_out : xbsIndex_r4/Reinterpret  force_arith_type=on  arith_type=Unsigned  force_bin_pt=on  bin_pt=0  block_type=reinterpret
  split : Subsystem  AncestorBlock=casper_library_flow_control/bus_expand  mask(bus_expand){mode=divisions of arbitrary size, outputNum=1, outputWidth=[32 32 32 32], outputBinaryPt=[0 0 0 0], outputArithmeticType=[0 0 0 0], show_format=off, outputToWorkspace=off, variablePrefix=out, outputToModelAsWell=on}
      mask prompts: outputNum "Number of outputs:"; outputWidth "Output width [msb ... lsb]:"; outputBinaryPt "Output binary point position [msb ... lsb]:"; outputArithmeticType "Output arithmetic type (ufix=0, fix=1, bool=2) [msb ... lsb]:"; show_format "Print format string?"; outputToWorkspace "Output to workspace?"; variablePrefix "Variable name prefix:"; outputToModelAsWell "Output to model as well?"
      mask help: Expands a 'bus' made using a bus_create or Xilinx concat block. The input will be divided into the specified number of outputs with the specified arithmetic types. Divisions are made from most significant bit.
      mask init:
      | bus_expand_init(gcb,...
      |     'mode', mode, ...
      |     'outputNum', outputNum, ...
      |     'outputWidth', outputWidth, ...
      |     'outputBinaryPt', outputBinaryPt, ...
      |     'outputArithmeticType', outputArithmeticType, ...
      |     'show_format', show_format, ...
      |     'outputToWorkspace', outputToWorkspace, ...
      |     'variablePrefix', variablePrefix, ...
      |     'outputToModelAsWell', outputToModelAsWell);
  dout : Outport
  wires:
  reinterpret_out/1 -> dout/1
  din/1 -> reinterpret/1
  reinterpret/1 -> split/1(bus_in)
  join/1(bus_out) -> reinterpret_out/1
  split/4(lsb_out1) -> join/1(in1)
  split/3(out2) -> join/2(in2)
  split/2(out3) -> join/3(in3)
  split/1(msb_out4) -> join/4(in4)

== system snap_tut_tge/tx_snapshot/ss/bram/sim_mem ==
  addr : Inport
  data : Inport  Port=2
  we : Inport  Port=3
  Data Type Conversion : DataTypeConversion  OutDataTypeStr=single
  Data Type Conversion1 : DataTypeConversion  OutDataTypeStr=double
  Data Type Conversion2 : DataTypeConversion  OutDataTypeStr=boolean
  sfunc : M-S-Function  FunctionName=shared_bram_sim_sfunc  Parameters=depth_bits, latency, init_vals  mask{depth_bits=addr_width, latency=csp_latency, init_vals=init_vals}
      mask prompts: depth_bits "Depth (2^?):"; latency "Latency (>=1):"; init_vals "Initial values:"
  sim_addr : xbsIndex_r4/Gateway Out  inherit_from_input=off  hdl_port=off  rows=1  columns=1  UseAsDAC=off  DACChannel='1'  interface=None  automatic_assignment=on  address_offset=hex2dec('00')  intf_name=''  intf_description=''  timing_constraint=None  locs_specified=off  LOCs={}  io_standard={}  block_type=gatewayout
  sim_data : xbsIndex_r4/Gateway Out  inherit_from_input=off  hdl_port=off  rows=1  columns=1  UseAsDAC=off  DACChannel='1'  interface=None  automatic_assignment=on  address_offset=hex2dec('00')  intf_name=''  intf_description=''  timing_constraint=None  locs_specified=off  LOCs={}  io_standard={}  block_type=gatewayout
  sim_we : xbsIndex_r4/Gateway Out  inherit_from_input=off  hdl_port=off  rows=1  columns=1  UseAsDAC=off  DACChannel='1'  interface=None  automatic_assignment=on  address_offset=hex2dec('00')  intf_name=''  intf_description=''  timing_constraint=None  locs_specified=off  LOCs={}  io_standard={}  block_type=gatewayout
  data_out : Outport
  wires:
  addr/1 -> sim_addr/1
  data/1 -> sim_data/1
  we/1 -> sim_we/1
  sim_addr/1 -> Data Type Conversion/1
  sim_data/1 -> Data Type Conversion1/1
  sim_we/1 -> Data Type Conversion2/1
  Data Type Conversion/1 -> sfunc/1  "addr"
  Data Type Conversion1/1 -> sfunc/2  "data_in"
  Data Type Conversion2/1 -> sfunc/3  "we"
  sfunc/1 -> data_out/1  "output"

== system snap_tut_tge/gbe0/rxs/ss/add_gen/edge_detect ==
  in : Inport
  Delay : xbsIndex_r4/Delay  rst=off  infoeditControl=Selection of Reset will increase slice count due to use of real FFs and instead of SRLs  en=off  latency=1  reg_retiming=off  dbl_ovrd=off  block_type=delay
  Inverter : xbsIndex_r4/Inverter  en=off  latency=0  dbl_ovrd=off  block_type=inv
  edge_op : xbsIndex_r4/Logical  logical_function=XNOR  inputs=2  en=off  latency=0  precision=Full  arith_type=Unsigned  n_bits=8  bin_pt=2  align_bp=on  dbl_ovrd=off  block_type=logical
  out : Outport
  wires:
  Delay/1 -> edge_op/2
  in/1 -> Delay/1, Inverter/1
  edge_op/1 -> out/1
  Inverter/1 -> edge_op/1

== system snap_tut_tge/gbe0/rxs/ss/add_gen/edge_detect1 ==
  in : Inport
  Delay : xbsIndex_r4/Delay  rst=off  infoeditControl=Selection of Reset will increase slice count due to use of real FFs and instead of SRLs  en=off  latency=1  reg_retiming=off  dbl_ovrd=off  block_type=delay
  Inverter : xbsIndex_r4/Inverter  en=off  latency=0  dbl_ovrd=off  block_type=inv
  edge_op : xbsIndex_r4/Logical  logical_function=XNOR  inputs=2  en=off  latency=0  precision=Full  arith_type=Unsigned  n_bits=8  bin_pt=2  align_bp=on  dbl_ovrd=off  block_type=logical
  out : Outport
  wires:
  Inverter/1 -> edge_op/1
  edge_op/1 -> out/1
  in/1 -> Inverter/1, Delay/1
  Delay/1 -> edge_op/2
